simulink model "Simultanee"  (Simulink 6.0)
settings: Solver=ode45  StartTime=0  StopTime=3*t0  RelTol=1e-3
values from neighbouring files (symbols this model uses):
  beta = 0.95    [Constantes.m]    (also in ConstantesBck.m; ResCourV1.m = 1; ResCrV1.m = 1; ResEnerV1.m = 1)
  Cmem = 1E-6*Sm*(1-b)    (= 2.826e-08)    [Constantes.m]    (also in ConstantesBck.m = 3.14e-11; ImpedanceZtissus.m = 4e-08; Ztissus.m = 4e-08; CalculCharge.m = 1)
  N = [6,8,5,5,7,1,2,6,9,1,1,9,4,8,8,7]    [Constantes.m]    (also in ConstantesBck.m; ImpedanceZtissus.m = 100; Ztissus.m = 100; charge.m = N(:,2))
  rapportIE = 10    [Constantes.m]
  Rcan = 6.398E3*Sm*(1-b)    (= 180.80748)    [Constantes.m]    (also in ConstantesBck.m = 0.03454; ImpedanceZtissus.m = 44; Ztissus.m = 44)
  t0 = 2E-3    (= 0.002)    [Constantes.m]    (also in ConstantesBck.m = 0.001)
undefined symbols (not defined in the file or in its folder): ln
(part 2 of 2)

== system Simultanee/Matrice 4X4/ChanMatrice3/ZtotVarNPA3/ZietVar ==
  InZiet : Inport  Orientation=left  Port=1  LatchInput=off
  Constant{,1..2,4} (4 alike) : Constant
  Contrôleur : Stateflow chart  Orientation=left
  Divide{1..4} (4 alike) : Product  Inputs=*/  OutScaling=2^-10
  Rct : Fcn  Expr=u*(3147.77*(1/((1E6*abs(u))^0.7199)))*1000
  Sum : Sum  Inputs=|++
  Sum1 : Sum  Inputs=|++
  Zcpa : Subsystem
  Zw : Subsystem
  OutZiet : Outport  Orientation=left
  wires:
  Constant/1 -> Divide1/1
  Constant1/1 -> Divide2/1
  Constant2/1 -> Divide3/1
  Zcpa/1(OutZcpa) -> Divide3/2
  Zw/1(OutZw) -> Divide2/2
  Rct/1 -> Divide1/2
  Divide3/1 -> Sum/1
  Constant4/1 -> Divide4/1
  Divide2/1 -> Sum/2
  Sum/1 -> Sum1/1
  Divide1/1 -> Sum1/2
  Sum1/1 -> Divide4/2
  Contrôleur/2(temp) -> Rct/1, Zw/1(InZw), Zcpa/1(InZcpa)
  InZiet/1 -> Contrôleur/1(u)
  Contrôleur/1(y) -> OutZiet/1
  Divide4/1 -> Contrôleur/2(calc)

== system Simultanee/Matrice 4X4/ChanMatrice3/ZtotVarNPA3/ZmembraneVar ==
  InZmem : Inport  Orientation=left  Port=1  LatchInput=off
  Constant : Constant
  Constant1 : Constant
  Constant2 : Constant
  Contrôleur : Stateflow chart  Orientation=left
  Divide : Product  Inputs=*/  OutScaling=2^-10
  Divide1 : Product  Inputs=*/  OutScaling=2^-10
  Divide2 : Product  Inputs=*/  OutScaling=2^-10
  Gain : Gain  Gain=2
  Rext : Fcn  Expr=u*(1.6342*((abs(u)*1E6)^0.1267))*1E3
  Rint : Fcn  Expr=u*(1.6342*((abs(u)*1E6)^0.1267))*1E3/rapportIE
  Sum : Sum  Inputs=|++
  Sum1 : Sum  Inputs=|++
  Transfer Fcn : TransferFcn  Numerator=[Rcan]  Denominator=[Rcan*Cmem 1]
  OutZmem : Outport  Orientation=left
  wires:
  Gain/1 -> Transfer Fcn/1
  Transfer Fcn/1 -> Sum/1
  Sum/1 -> Divide/2
  Rext/1 -> Divide1/2
  Constant1/1 -> Divide/1
  Constant/1 -> Divide1/1
  Divide/1 -> Sum1/1
  Constant2/1 -> Divide2/1
  Sum1/1 -> Divide2/2
  Rint/1 -> Sum/2
  Divide1/1 -> Sum1/2
  Contrôleur/2(temp) -> Rext/1, Rint/1, Gain/1
  Divide2/1 -> Contrôleur/2(calc)
  InZmem/1 -> Contrôleur/1(u)
  Contrôleur/1(y) -> OutZmem/1

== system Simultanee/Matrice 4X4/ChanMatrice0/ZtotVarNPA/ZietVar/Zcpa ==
  InZcpa : Inport  Port=1  LatchInput=off
  Cdl : Fcn  Expr=u*1E9/(918.15-80.854*ln(abs(u)*1E6))
  Fcn : Fcn  Expr=u(1)^beta
  Integrator : Integrator
  OutZcpa : Outport
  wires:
  Integrator/1 -> Fcn/1
  InZcpa/1 -> Cdl/1
  Fcn/1 -> OutZcpa/1
  Cdl/1 -> Integrator/1

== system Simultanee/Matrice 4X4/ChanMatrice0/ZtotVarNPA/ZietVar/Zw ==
  InZw : Inport  Port=1  LatchInput=off
  Gain : Gain  Gain=2
  Integrator : Integrator
  Math Function : Math  Operator=sqrt
  Product : Product
  sigma : Fcn  Expr=(67202-0.0688*((1E6*abs(u))^2)-11.273*(1E6*abs(u)))
  OutZw : Outport
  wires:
  Integrator/1 -> Math Function/1
  InZw/1 -> sigma/1, Gain/1
  Math Function/1 -> Product/1
  sigma/1 -> Product/2
  Product/1 -> OutZw/1
  Gain/1 -> Integrator/1

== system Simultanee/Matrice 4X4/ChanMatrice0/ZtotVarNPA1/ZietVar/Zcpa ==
  InZcpa : Inport  Port=1  LatchInput=off
  Cdl : Fcn  Expr=u*1E9/(918.15-80.854*ln(abs(u)*1E6))
  Fcn : Fcn  Expr=u(1)^beta
  Integrator : Integrator
  OutZcpa : Outport
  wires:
  Integrator/1 -> Fcn/1
  InZcpa/1 -> Cdl/1
  Fcn/1 -> OutZcpa/1
  Cdl/1 -> Integrator/1

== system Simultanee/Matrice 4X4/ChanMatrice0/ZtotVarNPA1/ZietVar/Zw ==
  InZw : Inport  Port=1  LatchInput=off
  Gain : Gain  Gain=2
  Integrator : Integrator
  Math Function : Math  Operator=sqrt
  Product : Product
  sigma : Fcn  Expr=(67202-0.0688*((1E6*abs(u))^2)-11.273*(1E6*abs(u)))
  OutZw : Outport
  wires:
  Integrator/1 -> Math Function/1
  InZw/1 -> sigma/1, Gain/1
  Math Function/1 -> Product/1
  sigma/1 -> Product/2
  Product/1 -> OutZw/1
  Gain/1 -> Integrator/1

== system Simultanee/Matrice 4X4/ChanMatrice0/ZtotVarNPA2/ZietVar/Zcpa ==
  InZcpa : Inport  Port=1  LatchInput=off
  Cdl : Fcn  Expr=u*1E9/(918.15-80.854*ln(abs(u)*1E6))
  Fcn : Fcn  Expr=u(1)^beta
  Integrator : Integrator
  OutZcpa : Outport
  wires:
  Integrator/1 -> Fcn/1
  InZcpa/1 -> Cdl/1
  Fcn/1 -> OutZcpa/1
  Cdl/1 -> Integrator/1

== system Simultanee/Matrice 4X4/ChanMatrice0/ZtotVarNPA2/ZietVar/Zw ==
  InZw : Inport  Port=1  LatchInput=off
  Gain : Gain  Gain=2
  Integrator : Integrator
  Math Function : Math  Operator=sqrt
  Product : Product
  sigma : Fcn  Expr=(67202-0.0688*((1E6*abs(u))^2)-11.273*(1E6*abs(u)))
  OutZw : Outport
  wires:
  Integrator/1 -> Math Function/1
  InZw/1 -> sigma/1, Gain/1
  Math Function/1 -> Product/1
  sigma/1 -> Product/2
  Product/1 -> OutZw/1
  Gain/1 -> Integrator/1

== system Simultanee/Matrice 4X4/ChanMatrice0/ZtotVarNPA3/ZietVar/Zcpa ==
  InZcpa : Inport  Port=1  LatchInput=off
  Cdl : Fcn  Expr=u*1E9/(918.15-80.854*ln(abs(u)*1E6))
  Fcn : Fcn  Expr=u(1)^beta
  Integrator : Integrator
  OutZcpa : Outport
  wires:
  Integrator/1 -> Fcn/1
  InZcpa/1 -> Cdl/1
  Fcn/1 -> OutZcpa/1
  Cdl/1 -> Integrator/1

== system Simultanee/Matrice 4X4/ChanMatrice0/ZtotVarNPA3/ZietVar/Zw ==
  InZw : Inport  Port=1  LatchInput=off
  Gain : Gain  Gain=2
  Integrator : Integrator
  Math Function : Math  Operator=sqrt
  Product : Product
  sigma : Fcn  Expr=(67202-0.0688*((1E6*abs(u))^2)-11.273*(1E6*abs(u)))
  OutZw : Outport
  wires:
  Integrator/1 -> Math Function/1
  InZw/1 -> sigma/1, Gain/1
  Math Function/1 -> Product/1
  sigma/1 -> Product/2
  Product/1 -> OutZw/1
  Gain/1 -> Integrator/1

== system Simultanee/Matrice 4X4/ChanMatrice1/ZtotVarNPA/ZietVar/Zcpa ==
  InZcpa : Inport  Port=1  LatchInput=off
  Cdl : Fcn  Expr=u*1E9/(918.15-80.854*ln(abs(u)*1E6))
  Fcn : Fcn  Expr=u(1)^beta
  Integrator : Integrator
  OutZcpa : Outport
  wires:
  Integrator/1 -> Fcn/1
  InZcpa/1 -> Cdl/1
  Fcn/1 -> OutZcpa/1
  Cdl/1 -> Integrator/1

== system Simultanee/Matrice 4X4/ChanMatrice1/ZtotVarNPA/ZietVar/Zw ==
  InZw : Inport  Port=1  LatchInput=off
  Gain : Gain  Gain=2
  Integrator : Integrator
  Math Function : Math  Operator=sqrt
  Product : Product
  sigma : Fcn  Expr=(67202-0.0688*((1E6*abs(u))^2)-11.273*(1E6*abs(u)))
  OutZw : Outport
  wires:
  Integrator/1 -> Math Function/1
  InZw/1 -> sigma/1, Gain/1
  Math Function/1 -> Product/1
  sigma/1 -> Product/2
  Product/1 -> OutZw/1
  Gain/1 -> Integrator/1

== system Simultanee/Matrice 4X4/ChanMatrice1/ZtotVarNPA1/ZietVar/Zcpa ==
  InZcpa : Inport  Port=1  LatchInput=off
  Cdl : Fcn  Expr=u*1E9/(918.15-80.854*ln(abs(u)*1E6))
  Fcn : Fcn  Expr=u(1)^beta
  Integrator : Integrator
  OutZcpa : Outport
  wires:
  Integrator/1 -> Fcn/1
  InZcpa/1 -> Cdl/1
  Fcn/1 -> OutZcpa/1
  Cdl/1 -> Integrator/1

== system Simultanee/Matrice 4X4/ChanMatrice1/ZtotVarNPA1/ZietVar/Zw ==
  InZw : Inport  Port=1  LatchInput=off
  Gain : Gain  Gain=2
  Integrator : Integrator
  Math Function : Math  Operator=sqrt
  Product : Product
  sigma : Fcn  Expr=(67202-0.0688*((1E6*abs(u))^2)-11.273*(1E6*abs(u)))
  OutZw : Outport
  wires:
  Integrator/1 -> Math Function/1
  InZw/1 -> sigma/1, Gain/1
  Math Function/1 -> Product/1
  sigma/1 -> Product/2
  Product/1 -> OutZw/1
  Gain/1 -> Integrator/1

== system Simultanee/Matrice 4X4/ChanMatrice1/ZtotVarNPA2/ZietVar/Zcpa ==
  InZcpa : Inport  Port=1  LatchInput=off
  Cdl : Fcn  Expr=u*1E9/(918.15-80.854*ln(abs(u)*1E6))
  Fcn : Fcn  Expr=u(1)^beta
  Integrator : Integrator
  OutZcpa : Outport
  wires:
  Integrator/1 -> Fcn/1
  InZcpa/1 -> Cdl/1
  Fcn/1 -> OutZcpa/1
  Cdl/1 -> Integrator/1

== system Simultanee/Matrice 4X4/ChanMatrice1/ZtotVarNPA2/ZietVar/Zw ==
  InZw : Inport  Port=1  LatchInput=off
  Gain : Gain  Gain=2
  Integrator : Integrator
  Math Function : Math  Operator=sqrt
  Product : Product
  sigma : Fcn  Expr=(67202-0.0688*((1E6*abs(u))^2)-11.273*(1E6*abs(u)))
  OutZw : Outport
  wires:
  Integrator/1 -> Math Function/1
  InZw/1 -> sigma/1, Gain/1
  Math Function/1 -> Product/1
  sigma/1 -> Product/2
  Product/1 -> OutZw/1
  Gain/1 -> Integrator/1

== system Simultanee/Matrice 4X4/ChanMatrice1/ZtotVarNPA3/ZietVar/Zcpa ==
  InZcpa : Inport  Port=1  LatchInput=off
  Cdl : Fcn  Expr=u*1E9/(918.15-80.854*ln(abs(u)*1E6))
  Fcn : Fcn  Expr=u(1)^beta
  Integrator : Integrator
  OutZcpa : Outport
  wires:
  Integrator/1 -> Fcn/1
  InZcpa/1 -> Cdl/1
  Fcn/1 -> OutZcpa/1
  Cdl/1 -> Integrator/1

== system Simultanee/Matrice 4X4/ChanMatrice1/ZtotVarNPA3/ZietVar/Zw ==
  InZw : Inport  Port=1  LatchInput=off
  Gain : Gain  Gain=2
  Integrator : Integrator
  Math Function : Math  Operator=sqrt
  Product : Product
  sigma : Fcn  Expr=(67202-0.0688*((1E6*abs(u))^2)-11.273*(1E6*abs(u)))
  OutZw : Outport
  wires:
  Integrator/1 -> Math Function/1
  InZw/1 -> sigma/1, Gain/1
  Math Function/1 -> Product/1
  sigma/1 -> Product/2
  Product/1 -> OutZw/1
  Gain/1 -> Integrator/1

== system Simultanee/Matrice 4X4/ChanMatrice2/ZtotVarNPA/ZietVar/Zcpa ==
  InZcpa : Inport  Port=1  LatchInput=off
  Cdl : Fcn  Expr=u*1E9/(918.15-80.854*ln(abs(u)*1E6))
  Fcn : Fcn  Expr=u(1)^beta
  Integrator : Integrator
  OutZcpa : Outport
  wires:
  Integrator/1 -> Fcn/1
  InZcpa/1 -> Cdl/1
  Fcn/1 -> OutZcpa/1
  Cdl/1 -> Integrator/1

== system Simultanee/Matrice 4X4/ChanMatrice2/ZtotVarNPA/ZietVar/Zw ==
  InZw : Inport  Port=1  LatchInput=off
  Gain : Gain  Gain=2
  Integrator : Integrator
  Math Function : Math  Operator=sqrt
  Product : Product
  sigma : Fcn  Expr=(67202-0.0688*((1E6*abs(u))^2)-11.273*(1E6*abs(u)))
  OutZw : Outport
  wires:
  Integrator/1 -> Math Function/1
  InZw/1 -> sigma/1, Gain/1
  Math Function/1 -> Product/1
  sigma/1 -> Product/2
  Product/1 -> OutZw/1
  Gain/1 -> Integrator/1

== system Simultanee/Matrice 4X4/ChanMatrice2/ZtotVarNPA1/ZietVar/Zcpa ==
  InZcpa : Inport  Port=1  LatchInput=off
  Cdl : Fcn  Expr=u*1E9/(918.15-80.854*ln(abs(u)*1E6))
  Fcn : Fcn  Expr=u(1)^beta
  Integrator : Integrator
  OutZcpa : Outport
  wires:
  Integrator/1 -> Fcn/1
  InZcpa/1 -> Cdl/1
  Fcn/1 -> OutZcpa/1
  Cdl/1 -> Integrator/1

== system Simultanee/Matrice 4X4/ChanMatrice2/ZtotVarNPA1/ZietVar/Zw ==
  InZw : Inport  Port=1  LatchInput=off
  Gain : Gain  Gain=2
  Integrator : Integrator
  Math Function : Math  Operator=sqrt
  Product : Product
  sigma : Fcn  Expr=(67202-0.0688*((1E6*abs(u))^2)-11.273*(1E6*abs(u)))
  OutZw : Outport
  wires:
  Integrator/1 -> Math Function/1
  InZw/1 -> sigma/1, Gain/1
  Math Function/1 -> Product/1
  sigma/1 -> Product/2
  Product/1 -> OutZw/1
  Gain/1 -> Integrator/1

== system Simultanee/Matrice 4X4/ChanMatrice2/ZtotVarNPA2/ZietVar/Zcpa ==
  InZcpa : Inport  Port=1  LatchInput=off
  Cdl : Fcn  Expr=u*1E9/(918.15-80.854*ln(abs(u)*1E6))
  Fcn : Fcn  Expr=u(1)^beta
  Integrator : Integrator
  OutZcpa : Outport
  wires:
  Integrator/1 -> Fcn/1
  InZcpa/1 -> Cdl/1
  Fcn/1 -> OutZcpa/1
  Cdl/1 -> Integrator/1

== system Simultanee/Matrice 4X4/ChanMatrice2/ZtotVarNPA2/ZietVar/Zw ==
  InZw : Inport  Port=1  LatchInput=off
  Gain : Gain  Gain=2
  Integrator : Integrator
  Math Function : Math  Operator=sqrt
  Product : Product
  sigma : Fcn  Expr=(67202-0.0688*((1E6*abs(u))^2)-11.273*(1E6*abs(u)))
  OutZw : Outport
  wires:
  Integrator/1 -> Math Function/1
  InZw/1 -> sigma/1, Gain/1
  Math Function/1 -> Product/1
  sigma/1 -> Product/2
  Product/1 -> OutZw/1
  Gain/1 -> Integrator/1

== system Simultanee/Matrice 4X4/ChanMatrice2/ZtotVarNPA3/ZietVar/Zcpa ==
  InZcpa : Inport  Port=1  LatchInput=off
  Cdl : Fcn  Expr=u*1E9/(918.15-80.854*ln(abs(u)*1E6))
  Fcn : Fcn  Expr=u(1)^beta
  Integrator : Integrator
  OutZcpa : Outport
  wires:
  Integrator/1 -> Fcn/1
  InZcpa/1 -> Cdl/1
  Fcn/1 -> OutZcpa/1
  Cdl/1 -> Integrator/1

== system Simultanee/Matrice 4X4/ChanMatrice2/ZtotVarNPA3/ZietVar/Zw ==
  InZw : Inport  Port=1  LatchInput=off
  Gain : Gain  Gain=2
  Integrator : Integrator
  Math Function : Math  Operator=sqrt
  Product : Product
  sigma : Fcn  Expr=(67202-0.0688*((1E6*abs(u))^2)-11.273*(1E6*abs(u)))
  OutZw : Outport
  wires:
  Integrator/1 -> Math Function/1
  InZw/1 -> sigma/1, Gain/1
  Math Function/1 -> Product/1
  sigma/1 -> Product/2
  Product/1 -> OutZw/1
  Gain/1 -> Integrator/1

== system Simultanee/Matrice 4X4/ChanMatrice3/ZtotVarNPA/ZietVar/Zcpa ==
  InZcpa : Inport  Port=1  LatchInput=off
  Cdl : Fcn  Expr=u*1E9/(918.15-80.854*ln(abs(u)*1E6))
  Fcn : Fcn  Expr=u(1)^beta
  Integrator : Integrator
  OutZcpa : Outport
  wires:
  Integrator/1 -> Fcn/1
  InZcpa/1 -> Cdl/1
  Fcn/1 -> OutZcpa/1
  Cdl/1 -> Integrator/1

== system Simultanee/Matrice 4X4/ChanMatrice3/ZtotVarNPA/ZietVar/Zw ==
  InZw : Inport  Port=1  LatchInput=off
  Gain : Gain  Gain=2
  Integrator : Integrator
  Math Function : Math  Operator=sqrt
  Product : Product
  sigma : Fcn  Expr=(67202-0.0688*((1E6*abs(u))^2)-11.273*(1E6*abs(u)))
  OutZw : Outport
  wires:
  Integrator/1 -> Math Function/1
  InZw/1 -> sigma/1, Gain/1
  Math Function/1 -> Product/1
  sigma/1 -> Product/2
  Product/1 -> OutZw/1
  Gain/1 -> Integrator/1

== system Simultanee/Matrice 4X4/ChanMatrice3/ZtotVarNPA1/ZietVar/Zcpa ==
  InZcpa : Inport  Port=1  LatchInput=off
  Cdl : Fcn  Expr=u*1E9/(918.15-80.854*ln(abs(u)*1E6))
  Fcn : Fcn  Expr=u(1)^beta
  Integrator : Integrator
  OutZcpa : Outport
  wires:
  Integrator/1 -> Fcn/1
  InZcpa/1 -> Cdl/1
  Fcn/1 -> OutZcpa/1
  Cdl/1 -> Integrator/1

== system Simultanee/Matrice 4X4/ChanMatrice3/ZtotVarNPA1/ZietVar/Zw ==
  InZw : Inport  Port=1  LatchInput=off
  Gain : Gain  Gain=2
  Integrator : Integrator
  Math Function : Math  Operator=sqrt
  Product : Product
  sigma : Fcn  Expr=(67202-0.0688*((1E6*abs(u))^2)-11.273*(1E6*abs(u)))
  OutZw : Outport
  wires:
  Integrator/1 -> Math Function/1
  InZw/1 -> sigma/1, Gain/1
  Math Function/1 -> Product/1
  sigma/1 -> Product/2
  Product/1 -> OutZw/1
  Gain/1 -> Integrator/1

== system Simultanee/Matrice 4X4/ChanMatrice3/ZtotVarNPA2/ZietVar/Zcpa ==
  InZcpa : Inport  Port=1  LatchInput=off
  Cdl : Fcn  Expr=u*1E9/(918.15-80.854*ln(abs(u)*1E6))
  Fcn : Fcn  Expr=u(1)^beta
  Integrator : Integrator
  OutZcpa : Outport
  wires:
  Integrator/1 -> Fcn/1
  InZcpa/1 -> Cdl/1
  Fcn/1 -> OutZcpa/1
  Cdl/1 -> Integrator/1

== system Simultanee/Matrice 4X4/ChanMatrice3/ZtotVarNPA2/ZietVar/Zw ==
  InZw : Inport  Port=1  LatchInput=off
  Gain : Gain  Gain=2
  Integrator : Integrator
  Math Function : Math  Operator=sqrt
  Product : Product
  sigma : Fcn  Expr=(67202-0.0688*((1E6*abs(u))^2)-11.273*(1E6*abs(u)))
  OutZw : Outport
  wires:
  Integrator/1 -> Math Function/1
  InZw/1 -> sigma/1, Gain/1
  Math Function/1 -> Product/1
  sigma/1 -> Product/2
  Product/1 -> OutZw/1
  Gain/1 -> Integrator/1

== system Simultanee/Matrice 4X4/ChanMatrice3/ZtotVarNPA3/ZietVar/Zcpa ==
  InZcpa : Inport  Port=1  LatchInput=off
  Cdl : Fcn  Expr=u*1E9/(918.15-80.854*ln(abs(u)*1E6))
  Fcn : Fcn  Expr=u(1)^beta
  Integrator : Integrator
  OutZcpa : Outport
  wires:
  Integrator/1 -> Fcn/1
  InZcpa/1 -> Cdl/1
  Fcn/1 -> OutZcpa/1
  Cdl/1 -> Integrator/1

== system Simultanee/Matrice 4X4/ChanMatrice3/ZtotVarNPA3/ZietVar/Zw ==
  InZw : Inport  Port=1  LatchInput=off
  Gain : Gain  Gain=2
  Integrator : Integrator
  Math Function : Math  Operator=sqrt
  Product : Product
  sigma : Fcn  Expr=(67202-0.0688*((1E6*abs(u))^2)-11.273*(1E6*abs(u)))
  OutZw : Outport
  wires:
  Integrator/1 -> Math Function/1
  InZw/1 -> sigma/1, Gain/1
  Math Function/1 -> Product/1
  sigma/1 -> Product/2
  Product/1 -> OutZw/1
  Gain/1 -> Integrator/1

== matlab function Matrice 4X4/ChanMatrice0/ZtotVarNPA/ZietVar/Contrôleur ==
function [y,temp] = fcn(u,calc)
% This block supports an embeddable subset of the MATLAB language.
% See the help menu for details. 

if u == 0
    y = 0;
    temp = 1E-6;
else
    y = calc;
    temp = u;
end

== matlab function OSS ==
function [S0,Ref0,S1,Ref1,S2,Ref2,S3,Ref3,S4,Ref4,S5,Ref5,S6,Ref6,S7,Ref7,S8,Ref8,S9,Ref9,S10,Ref10,S11,Ref11,S12,Ref12,S13,Ref13,S14,Ref14,S15,Ref15,MatCourant] = fcn(u0,u1,u2,u3,u4,u5,u6,u7,u8,u9,u10,u11,u12,u13,u14,u15,tc0,tc1,tc2,dyn,rst)
%Fonction qui détermine les endroits à stimuler pour obtenir une puissance 
%moyenne par canal minimal

%Valeur utilisée
Vdd=3.3;
Imax=200E-6;

%Initialisation des tableaux de sorties
SOut=[0,0,0,0,0,0,0,0,0,0,0,0,0,0,0,0];

%Détermination des sorties actives
Signe = 1;
if(tc0==0)
    Signe=-1;
else
    Signe=1;
end

RefOut=0;
if not(rst == 0)
    SOut(1)=u0*Imax/10*Signe;
    SOut(2)=u1*Imax/10*Signe;
    SOut(3)=u2*Imax/10*Signe;
    SOut(4)=u3*Imax/10*Signe;
    SOut(5)=u4*Imax/10*Signe;
    SOut(6)=u5*Imax/10*Signe;
    SOut(7)=u6*Imax/10*Signe;
    SOut(8)=u7*Imax/10*Signe;
    SOut(9)=u8*Imax/10*Signe;
    SOut(10)=u9*Imax/10*Signe;
    SOut(11)=u10*Imax/10*Signe;
    SOut(12)=u11*Imax/10*Signe;
    SOut(13)=u12*Imax/10*Signe;
    SOut(14)=u13*Imax/10*Signe;
    SOut(15)=u14*Imax/10*Signe;
    SOut(16)=u15*Imax/10*Signe;
end

%Assignation des sorties
S0=SOut(1);
Ref0=RefOut;
S1=SOut(2);
Ref1=RefOut;
S2=SOut(3);
Ref2=RefOut;
S3=SOut(4);
Ref3=RefOut;
S4=SOut(5);
Ref4=RefOut;
S5=SOut(6);
Ref5=RefOut;
S6=SOut(7);
Ref6=RefOut;
S7=SOut(8);
Ref7=RefOut;
S8=SOut(9);
Ref8=RefOut;
S9=SOut(10);
Ref9=RefOut;
S10=SOut(11);
Ref10=RefOut;
S11=SOut(12);
Ref11=RefOut;
S12=SOut(13);
Ref12=RefOut;
S13=SOut(14);
Ref13=RefOut;
S14=SOut(15);
Ref14=RefOut;
S15=SOut(16);
Ref15=RefOut;
MatCourant=SOut;

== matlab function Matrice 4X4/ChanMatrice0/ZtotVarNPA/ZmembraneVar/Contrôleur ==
function [y,temp] = fcn(u,calc)
% This block supports an embeddable subset of the MATLAB language.
% See the help menu for details. 

if u == 0
    y = 0;
    temp = 1E-6;
else
    y = calc;
    temp = u;
end

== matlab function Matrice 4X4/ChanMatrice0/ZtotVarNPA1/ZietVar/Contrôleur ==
function [y,temp] = fcn(u,calc)
% This block supports an embeddable subset of the MATLAB language.
% See the help menu for details. 

if u == 0
    y = 0;
    temp = 1E-6;
else
    y = calc;
    temp = u;
end

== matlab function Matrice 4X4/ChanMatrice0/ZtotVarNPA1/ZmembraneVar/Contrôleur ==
function [y,temp] = fcn(u,calc)
% This block supports an embeddable subset of the MATLAB language.
% See the help menu for details. 

if u == 0
    y = 0;
    temp = 1E-6;
else
    y = calc;
    temp = u;
end

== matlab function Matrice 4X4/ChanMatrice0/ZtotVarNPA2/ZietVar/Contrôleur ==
function [y,temp] = fcn(u,calc)
% This block supports an embeddable subset of the MATLAB language.
% See the help menu for details. 

if u == 0
    y = 0;
    temp = 1E-6;
else
    y = calc;
    temp = u;
end

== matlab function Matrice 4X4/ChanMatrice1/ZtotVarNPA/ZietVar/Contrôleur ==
function [y,temp] = fcn(u,calc)
% This block supports an embeddable subset of the MATLAB language.
% See the help menu for details. 

if u == 0
    y = 0;
    temp = 1E-6;
else
    y = calc;
    temp = u;
end

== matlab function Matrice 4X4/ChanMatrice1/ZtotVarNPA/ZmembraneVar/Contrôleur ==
function [y,temp] = fcn(u,calc)
% This block supports an embeddable subset of the MATLAB language.
% See the help menu for details. 

if u == 0
    y = 0;
    temp = 1E-6;
else
    y = calc;
    temp = u;
end

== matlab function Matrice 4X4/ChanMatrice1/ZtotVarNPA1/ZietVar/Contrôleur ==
function [y,temp] = fcn(u,calc)
% This block supports an embeddable subset of the MATLAB language.
% See the help menu for details. 

if u == 0
    y = 0;
    temp = 1E-6;
else
    y = calc;
    temp = u;
end

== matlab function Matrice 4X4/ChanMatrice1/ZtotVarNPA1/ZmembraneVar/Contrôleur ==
function [y,temp] = fcn(u,calc)
% This block supports an embeddable subset of the MATLAB language.
% See the help menu for details. 

if u == 0
    y = 0;
    temp = 1E-6;
else
    y = calc;
    temp = u;
end

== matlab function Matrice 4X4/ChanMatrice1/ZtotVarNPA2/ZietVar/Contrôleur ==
function [y,temp] = fcn(u,calc)
% This block supports an embeddable subset of the MATLAB language.
% See the help menu for details. 

if u == 0
    y = 0;
    temp = 1E-6;
else
    y = calc;
    temp = u;
end

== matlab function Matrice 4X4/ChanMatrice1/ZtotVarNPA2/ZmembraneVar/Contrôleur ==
function [y,temp] = fcn(u,calc)
% This block supports an embeddable subset of the MATLAB language.
% See the help menu for details. 

if u == 0
    y = 0;
    temp = 1E-6;
else
    y = calc;
    temp = u;
end

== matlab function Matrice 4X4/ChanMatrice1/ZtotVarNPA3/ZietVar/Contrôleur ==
function [y,temp] = fcn(u,calc)
% This block supports an embeddable subset of the MATLAB language.
% See the help menu for details. 

if u == 0
    y = 0;
    temp = 1E-6;
else
    y = calc;
    temp = u;
end

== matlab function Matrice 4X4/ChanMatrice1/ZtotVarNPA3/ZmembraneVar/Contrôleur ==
function [y,temp] = fcn(u,calc)
% This block supports an embeddable subset of the MATLAB language.
% See the help menu for details. 

if u == 0
    y = 0;
    temp = 1E-6;
else
    y = calc;
    temp = u;
end

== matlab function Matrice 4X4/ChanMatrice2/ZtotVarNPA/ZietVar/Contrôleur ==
function [y,temp] = fcn(u,calc)
% This block supports an embeddable subset of the MATLAB language.
% See the help menu for details. 

if u == 0
    y = 0;
    temp = 1E-6;
else
    y = calc;
    temp = u;
end

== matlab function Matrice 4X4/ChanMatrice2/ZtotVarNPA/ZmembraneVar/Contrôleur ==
function [y,temp] = fcn(u,calc)
% This block supports an embeddable subset of the MATLAB language.
% See the help menu for details. 

if u == 0
    y = 0;
    temp = 1E-6;
else
    y = calc;
    temp = u;
end

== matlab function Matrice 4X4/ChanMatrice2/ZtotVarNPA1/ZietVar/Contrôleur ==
function [y,temp] = fcn(u,calc)
% This block supports an embeddable subset of the MATLAB language.
% See the help menu for details. 

if u == 0
    y = 0;
    temp = 1E-6;
else
    y = calc;
    temp = u;
end

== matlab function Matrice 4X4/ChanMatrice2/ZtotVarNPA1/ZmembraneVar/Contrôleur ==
function [y,temp] = fcn(u,calc)
% This block supports an embeddable subset of the MATLAB language.
% See the help menu for details. 

if u == 0
    y = 0;
    temp = 1E-6;
else
    y = calc;
    temp = u;
end

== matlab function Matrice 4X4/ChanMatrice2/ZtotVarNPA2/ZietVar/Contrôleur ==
function [y,temp] = fcn(u,calc)
% This block supports an embeddable subset of the MATLAB language.
% See the help menu for details. 

if u == 0
    y = 0;
    temp = 1E-6;
else
    y = calc;
    temp = u;
end

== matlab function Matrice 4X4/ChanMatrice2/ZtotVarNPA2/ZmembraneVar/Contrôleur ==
function [y,temp] = fcn(u,calc)
% This block supports an embeddable subset of the MATLAB language.
% See the help menu for details. 

if u == 0
    y = 0;
    temp = 1E-6;
else
    y = calc;
    temp = u;
end

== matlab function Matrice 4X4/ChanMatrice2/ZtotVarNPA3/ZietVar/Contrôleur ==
function [y,temp] = fcn(u,calc)
% This block supports an embeddable subset of the MATLAB language.
% See the help menu for details. 

if u == 0
    y = 0;
    temp = 1E-6;
else
    y = calc;
    temp = u;
end

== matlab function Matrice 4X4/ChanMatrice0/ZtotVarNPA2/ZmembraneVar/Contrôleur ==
function [y,temp] = fcn(u,calc)
% This block supports an embeddable subset of the MATLAB language.
% See the help menu for details. 

if u == 0
    y = 0;
    temp = 1E-6;
else
    y = calc;
    temp = u;
end

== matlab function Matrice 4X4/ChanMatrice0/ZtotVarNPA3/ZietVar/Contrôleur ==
function [y,temp] = fcn(u,calc)
% This block supports an embeddable subset of the MATLAB language.
% See the help menu for details. 

if u == 0
    y = 0;
    temp = 1E-6;
else
    y = calc;
    temp = u;
end

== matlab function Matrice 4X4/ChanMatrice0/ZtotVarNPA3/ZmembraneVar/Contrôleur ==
function [y,temp] = fcn(u,calc)
% This block supports an embeddable subset of the MATLAB language.
% See the help menu for details. 

if u == 0
    y = 0;
    temp = 1E-6;
else
    y = calc;
    temp = u;
end

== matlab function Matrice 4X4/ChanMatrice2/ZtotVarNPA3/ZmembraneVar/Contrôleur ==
function [y,temp] = fcn(u,calc)
% This block supports an embeddable subset of the MATLAB language.
% See the help menu for details. 

if u == 0
    y = 0;
    temp = 1E-6;
else
    y = calc;
    temp = u;
end

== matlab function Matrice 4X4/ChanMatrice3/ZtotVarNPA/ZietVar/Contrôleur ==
function [y,temp] = fcn(u,calc)
% This block supports an embeddable subset of the MATLAB language.
% See the help menu for details. 

if u == 0
    y = 0;
    temp = 1E-6;
else
    y = calc;
    temp = u;
end

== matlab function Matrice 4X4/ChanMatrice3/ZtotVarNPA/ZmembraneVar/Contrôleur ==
function [y,temp] = fcn(u,calc)
% This block supports an embeddable subset of the MATLAB language.
% See the help menu for details. 

if u == 0
    y = 0;
    temp = 1E-6;
else
    y = calc;
    temp = u;
end

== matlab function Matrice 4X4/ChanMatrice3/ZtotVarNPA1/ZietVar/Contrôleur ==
function [y,temp] = fcn(u,calc)
% This block supports an embeddable subset of the MATLAB language.
% See the help menu for details. 

if u == 0
    y = 0;
    temp = 1E-6;
else
    y = calc;
    temp = u;
end

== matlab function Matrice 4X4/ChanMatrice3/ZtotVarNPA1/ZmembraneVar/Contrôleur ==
function [y,temp] = fcn(u,calc)
% This block supports an embeddable subset of the MATLAB language.
% See the help menu for details. 

if u == 0
    y = 0;
    temp = 1E-6;
else
    y = calc;
    temp = u;
end

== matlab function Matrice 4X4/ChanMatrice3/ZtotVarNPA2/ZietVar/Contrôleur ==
function [y,temp] = fcn(u,calc)
% This block supports an embeddable subset of the MATLAB language.
% See the help menu for details. 

if u == 0
    y = 0;
    temp = 1E-6;
else
    y = calc;
    temp = u;
end

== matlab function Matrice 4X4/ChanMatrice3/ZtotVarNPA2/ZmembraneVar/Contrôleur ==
function [y,temp] = fcn(u,calc)
% This block supports an embeddable subset of the MATLAB language.
% See the help menu for details. 

if u == 0
    y = 0;
    temp = 1E-6;
else
    y = calc;
    temp = u;
end

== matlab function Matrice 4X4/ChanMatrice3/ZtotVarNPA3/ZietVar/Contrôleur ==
function [y,temp] = fcn(u,calc)
% This block supports an embeddable subset of the MATLAB language.
% See the help menu for details. 

if u == 0
    y = 0;
    temp = 1E-6;
else
    y = calc;
    temp = u;
end

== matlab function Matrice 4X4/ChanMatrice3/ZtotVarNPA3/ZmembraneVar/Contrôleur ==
function [y,temp] = fcn(u,calc)
% This block supports an embeddable subset of the MATLAB language.
% See the help menu for details. 

if u == 0
    y = 0;
    temp = 1E-6;
else
    y = calc;
    temp = u;
end
